PROGRAM MAIN
VAR
	bCONNECT: BOOL;
	bCreatCMD: BOOL;
	bExecute : BOOL;
	bDISCONNECT: BOOL;
			
	R_TRIG1: R_TRIG;	
	R_TRIG2: R_TRIG;
	R_TRIG3: R_TRIG;
	R_TRIG4: R_TRIG;
		
	nState: INT;
	nState_Connect: INT;
	nState_Disconnect: INT;
	
	bConn: BOOL;
	bSP: BOOL;	
	bResult: BOOL;
	bData: BOOL;
		
	nDBID: UDINT := 1;
	
	fbSQLDatabase: FB_SQLDatabase(sNetID:='', tTimeout:=T#10S);
	fbSqlCommand : FB_SQLCommand(sNetID := '', tTimeout := T#10S);
	
	
	ipResultEvent : Tc3_Eventlogger.I_TcResultEvent;
	bError : BOOL;
	sErrorClass : WSTRING(255);
	sErrorMsg : WSTRING(255);
	sCmd: STRING(INT#110);
END_VAR

R_TRIG1(CLK:=bCONNECT);
IF R_TRIG1.Q AND nState = 0 THEN
	bCONNECT := FALSE;
	nState := 1;
END_IF	

R_TRIG2(CLK:=bCreatCMD);
IF R_TRIG2.Q AND nState = 0 THEN
	bCreatCMD := FALSE;
	nState := 2;
END_IF	

R_TRIG3(CLK:=bExecute);
IF R_TRIG3.Q AND nState = 0 THEN
	bExecute := FALSE; 
	nState := 3;
END_IF

R_TRIG4(CLK:=bDISCONNECT);
IF R_TRIG4.Q THEN
	bDISCONNECT := FALSE;
	nState := 4;
END_IF

CASE nState OF
	0:(*Idle*)
		;
	1: // Connect to database and create stored procedure instance 
		IF fbSQLDatabase.Connect(hDBID:= nDBID) THEN
					ipResultEvent := fbSQLDatabase.ipTcResultEvent;
					bConn := NOT fbSQLDatabase.bError;
					IF bConn THEN
						nState:=0;;
					ELSE
						nState:=200;
					END_IF
				END_IF 
				
	2: // create a command reference
		IF fbSqlDatabase.CreateCmd(ADR(fbSqlCommand)) THEN
			IF fbSqlDatabase.bError THEN
				nState := 200; 
			ELSE
				nState := 0; 
			END_IF
		END_IF
		
	3:	// you can generate this with the SQL Query Editor 
		sCmd := 'INSERT INTO Mytest_table (ID, Timestamp, Name, Value) VALUES (1, $'2018-01-31 14:59:27$', $'Temperature$', 21.3)';

		// call sql command
		IF fbSQLCommand.Execute(ADR(sCmd), SIZEOF(sCmd)) THEN
			IF fbSQLCommand.bError THEN
				nState := 255; 
			ELSE
				nState := 0; 
			END_IF
		END_IF
	4:// Disconnect all
		CASE nState_Disconnect OF
			0:
				IF bConn THEN
					IF fbSQLDatabase.Disconnect() THEN
						nState_Disconnect := 1;
					END_IF
				ELSE
					nState_Disconnect := 1;
				END_IF
			1:
				bData := FALSE;
				bSP := FALSE;
				bConn := FALSE;
				bResult := FALSE;
				sErrorClass := "";
				sErrorMsg := "";
				bError := FALSE;
				nState_Disconnect := 0;
				nState := 0;
		END_CASE
	200:
		bError := ipResultEvent.Severity = E_Severity.Error;
		sErrorClass := ipResultEvent.EventClassDisplayName;
		sErrorMsg := ipResultEvent.Text;
		nState := 0;
END_CASE

END_PROGRAM
